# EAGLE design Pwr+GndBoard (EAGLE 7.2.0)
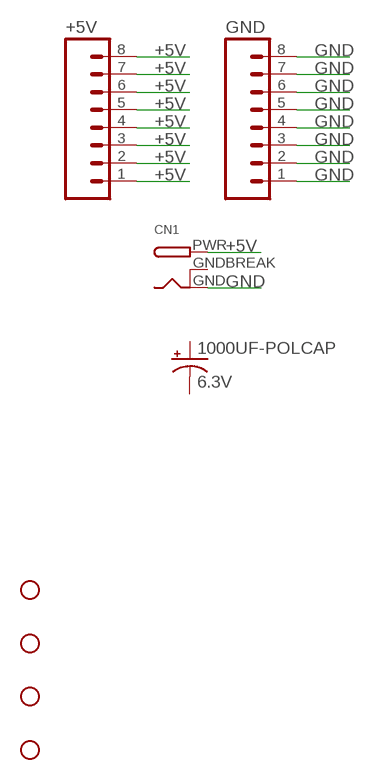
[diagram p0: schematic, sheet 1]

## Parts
1000UF-POLCAP  6.3V  CAP_POLPTH4  [CPOL-RADIAL-1000UF-25V]
+5V  M08LONGPADS  [1X08_LONGPADS]
CN1  DCBARRELPTH  [DCJACK_2MM_PTH]
GND  M08LONGPADS  [1X08_LONGPADS]
JP2  STAND-OFF  [STAND-OFF]
JP3  STAND-OFF  [STAND-OFF]
JP4  STAND-OFF  [STAND-OFF]
JP5  STAND-OFF  [STAND-OFF]

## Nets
+5V: +5V.1 +5V.2 +5V.3 +5V.4 +5V.5 +5V.6 +5V.7 +5V.8 CN1.PWR
GND: CN1.GND GND.1 GND.2 GND.3 GND.4 GND.5 GND.6 GND.7 GND.8
Unconnected: 1000UF-POLCAP.1(+) 1000UF-POLCAP.2(-)

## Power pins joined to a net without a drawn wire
GNDBREAK: CN1.GNDBREAK

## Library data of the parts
1000UF-POLCAP = 01_SparkFun:CAP_POL: Capacitor Polarized
+5V GND = 01_SparkFun:M08: Header 8 Standard 8-pin 0.1" header. Use with straight break away headers (SKU : PRT-00116), right angle break away headers (PRT-00553), swiss pins (PRT-00743), machine pins (PRT-00117), and female headers (PRT-00115).
CN1 = adafruit:DCBARREL: 2.0mm DC Barrel Jack DCJACK_2MM_PTH - Through Hole Jack (4UConnector: 05537)
JP2-JP5 = 01_SparkFun:STAND-OFF: Stand Off

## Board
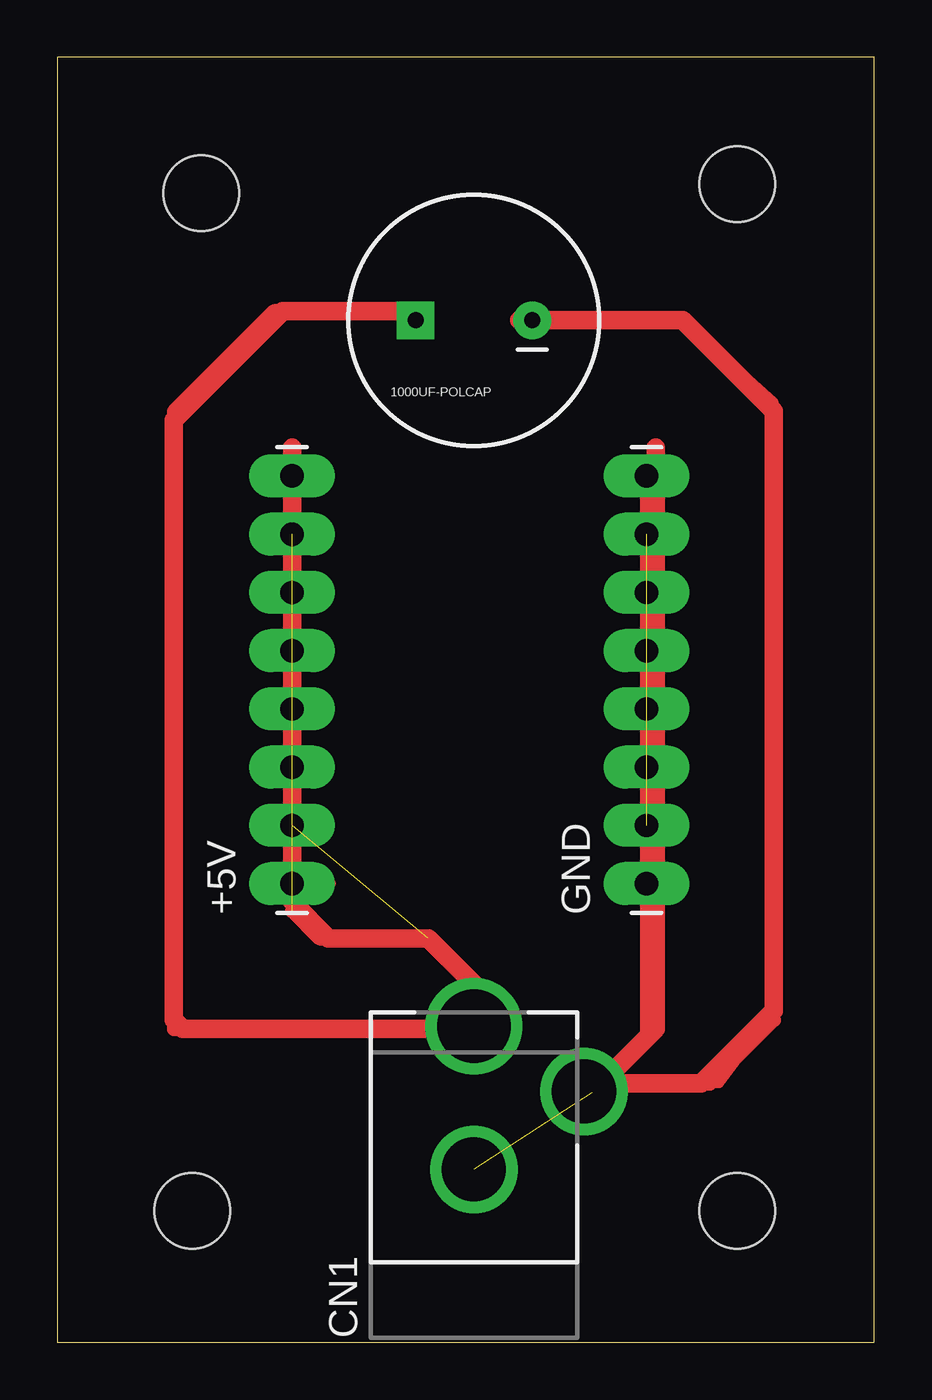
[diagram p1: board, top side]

Size 35.62 x 56.03 mm. Coordinates in mm from the lower left corner, seen from the top.
Outline: 0,0 35.62,0 35.62,56.03 0,56.03 0,0
Copper layers (1*16): Top 0.035mm / dielectric 1.5mm / Bottom 0.035mm
Design rules "default": minimum track width 10mil, minimum drill 24mil, track to track 8mil, track to pad 8mil, pad to pad 8mil, via to via 8mil, smd to smd 8mil, copper to edge 40mil, drill to drill 8mil, minimum pad ring 10mil, minimum via ring 8mil, stop-mask expansion 4mil, vias tented up to drill 0mil, thermal gap 10mil

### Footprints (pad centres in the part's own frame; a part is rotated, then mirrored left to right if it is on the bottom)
CPOL-RADIAL-1000UF-25V = drill 0.7 pad 1.651 square: 1 2.54,0 | drill 0.7 pad 1.651: 2 -2.54,0
1X08_LONGPADS = drill 1.016 pad 1.88 long: 1 0,0; 2 2.54,0; 3 5.08,0; 4 7.62,0; 5 10.16,0; 6 12.7,0; 7 15.24,0; 8 17.78,0
DCJACK_2MM_PTH = drill 2.8: GND 0,7.35; GNDBREAK 4.8,10.75 | drill 3.2: PWR 0,13.6
STAND-OFF = hole 3.302: 0,0

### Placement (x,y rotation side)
1000UF-POLCAP  18.16,44.56 180 top
+5V  10.23,19.99 90 top
CN1  18.16,0.18 0 top
GND  25.68,19.99 90 top
JP2  5.87,5.73 0 top
JP3  29.65,5.73 0 top
JP4  29.65,50.51 0 top
JP5  6.27,50.11 0 top

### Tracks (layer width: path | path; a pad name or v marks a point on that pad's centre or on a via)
+5V  (7 unrouted)
  Top 0.406: +5V.8 +5V.1 | +5V.1 11.94,20 | CN1.PWR 18.16,15.64 | 12.61,17.62 12.21,17.62 | +5V.1 10.23,18.81
  Top 0.61: 18.16,15.64 16.17,17.62 12.61,17.62 | 10.23,18.81 11.42,17.62 11.82,17.62 12.21,17.62 | +5V.8 10.23,18.81 | 10.23,18.81 | 15.38,44.96 9.44,44.96 5.08,40.6 5.08,40.2 | 18.55,13.66 5.48,13.66 5.08,13.66 5.08,14.05
  Top 0.813: 15.38,44.96 9.83,44.96 5.08,40.2 5.08,14.05 5.48,13.66 18.16,13.66 18.55,14.05 18.55,15.24 16.17,17.62 11.82,17.62 10.23,19.2 10.23,39.01
GND  (7 unrouted)
  Top 0.406: GND.8 GND.1 25.68,13.26
  Top 0.61: GND.8 25.68,13.26 23.31,10.88
N$1
  Top 0.406: 27.27,44.56 31.23,41 31.23,40.6 | 31.23,14.45 28.85,11.28 23.7,11.28 | 23.31,11.28 22.91,11.28 22.51,10.88
  Top 0.61: 20.93,44.56 27.27,44.56 | 23.31,11.28 23.7,11.28 28.46,11.28 31.23,14.05 31.23,14.45 31.23,40.6 30.44,41.39
  Top 0.813: 26.08,39.01 26.08,13.66 23.7,11.28 28.06,11.28 31.23,14.45 31.23,40.6 27.27,44.56 20.14,44.56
